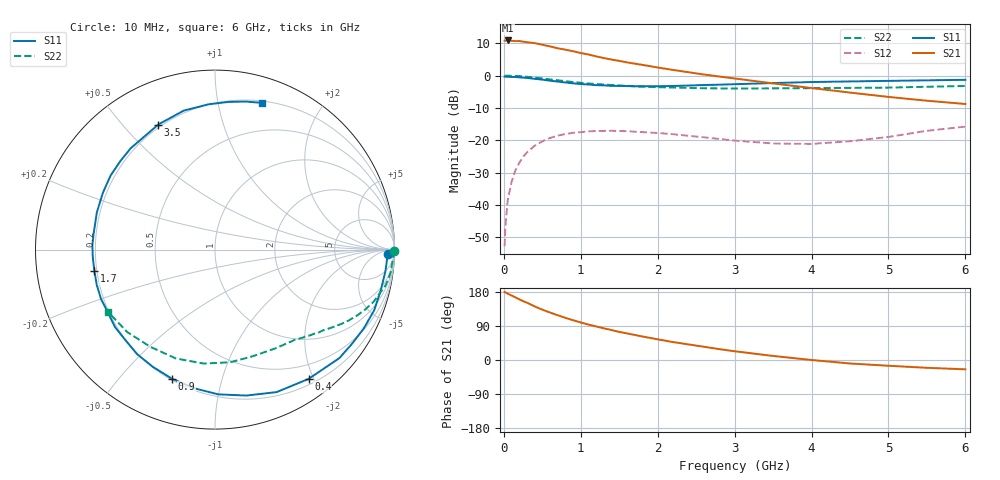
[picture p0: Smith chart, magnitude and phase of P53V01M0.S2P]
! SIEMENS Small Signal Semiconductors
! BFP183
! Si NPN RF Bipolar Junction Transistor in SOT143
! VCE = 3 V  IC = 1 mA
! Common Emitter S-Parameters:  March  1996
# GHz  S  MA  R  50
!  f  S11  S21  S12  S22
! GHz  MAG  ANG  MAG  ANG  MAG  ANG  MAG  ANG
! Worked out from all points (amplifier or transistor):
!   36 points, 10 MHz to 6 GHz, reference 50 ohm
!   highest |S21| = 10.8 dB at 50 MHz (marker M1)
!   |S21| within 3 dB of that: start of sweep to 829.9 MHz
!   unconditionally stable (mu >= 1): 2.476 GHz to end of sweep
!   at 250 MHz: K = 0.10, MSG = 17.8 dB, |S12| = -25.2 dB
!   at 1.4 GHz: K = 0.55, MSG = 11.0 dB, |S12| = -17.1 dB
!   at 6 GHz: K = 1.06, MAG = 2.0 dB, |S12| = -15.8 dB
!   S11 on the Smith chart (normalised r, x): 10 MHz: 36, -26; 400 MHz: 0.28, -1.93; 900 MHz: 0.21, -0.70; 1.7 GHz: 0.19, -0.09; 3.5 GHz: 0.19, +0.63; 6 GHz: 0.22, +1.35
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0.01  0.9647 -1.5  3.464 179.3  0.0023 93.5  0.9999 -0.5
0.02  0.9603 -3.0  3.451 178.7  0.0046 87.6  0.9926 -1.0
0.05  0.9574 -7.1  3.486 175.1  0.0117 87.0  0.9951 -2.4
0.1  0.9513 -13.8  3.442 170.2  0.0225 80.7  0.9888 -4.9
0.15  0.9491 -20.9  3.406 165.2  0.0341 77.1  0.9871 -7.3
0.2  0.9382 -27.9  3.417 160.1  0.0446 73.2  0.9795 -9.7
0.4  0.8893 -54.1  3.172 141.5  0.082 57.8  0.9311 -18.1
0.5  0.865 -66.6  2.996 132.9  0.0961 50.2  0.9005 -21.8
0.6  0.8319 -77.8  2.823 125.3  0.1083 44.2  0.8715 -25.0
0.7  0.8068 -88.7  2.639 118.1  0.1176 38.7  0.8442 -27.8
0.9  0.758 -108.5  2.374 105.0  0.13 28.9  0.7937 -32.6
1.1  0.7264 -126.7  2.113 93.4  0.1371 20.8  0.7529 -36.6
1.3  0.7047 -142.3  1.862 83.6  0.1394 13.8  0.7253 -40.2
1.5  0.692 -156.6  1.685 74.1  0.1386 8.4  0.7012 -43.4
1.7  0.6825 -169.8  1.529 66.2  0.1355 3.7  0.6813 -46.9
1.9  0.6837 178.1  1.396 58.4  0.1313 0.0  0.6664 -50.1
2.2  0.6902 162.5  1.22 47.3  0.1238 -4.2  0.6515 -55.2
2.8  0.722 136.9  0.966 28.7  0.1046 -6.6  0.6322 -66.8
3.5  0.7652 114.4  0.755 10.7  0.089 0.3  0.6335 -82.3
4.5  0.8104 92.5  0.545 -9.2  0.0963 19.5  0.6445 -109.8
5.5  0.843 78.0  0.408 -20.6  0.1398 26.5  0.6708 -136.7
6  0.8588 72.1  0.363 -24.6  0.1622 23.6  0.689 -149.5
